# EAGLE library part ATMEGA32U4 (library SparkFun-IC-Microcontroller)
Atmel MCU, 32KByte Atmel 44-pin 8-bit Microcontroller with 32KBytes of ISP Flash and USB Controller Datasheet SparkFun Products LilyPad Arduino USB - ATmega32U4 Board (DEV-12049) Pro Micro - 5V/16MHz (DEV-12640) Pro Micro - 3.3V/8MHz (DEV-12587) Fio v3 - ATmega32U4 (DEV-11520) Qduino Mini (DEV-13614) Makey Makey - Standard Kit (WIG-11511) Makey Makey Deluxe Kit (WIG-11519)
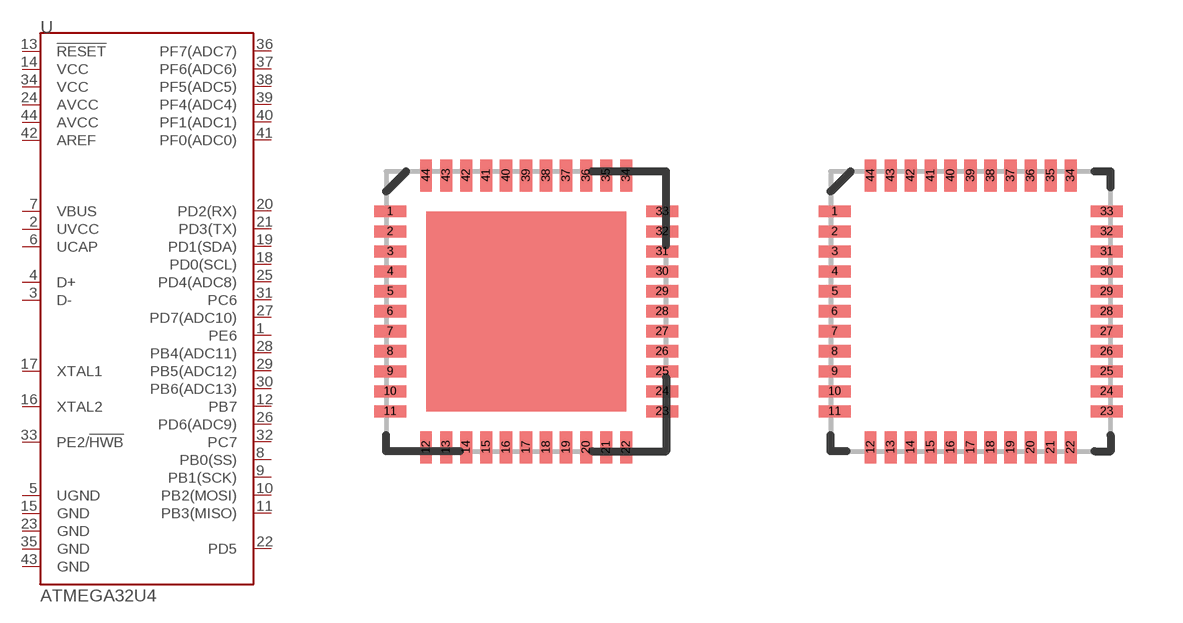
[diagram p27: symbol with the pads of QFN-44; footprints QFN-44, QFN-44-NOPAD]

Designator prefix U

## ATMEGA32U4QFN (PROD_ID: IC-10828; VALUE: 32U4)  [QFN-44]
1  PE6
2  UVCC
3  D-
4  D+
5  UGND
6  UCAP
7  VBUS
8  PB0(SS)
9  PB1(SCK)
10  PB2(MOSI)
11  PB3(MISO)
12  PB7
13  !RESET
14  VCC
15  GND
16  XTAL2
17  XTAL1
18  PD0(SCL)
19  PD1(SDA)
20  PD2(RX)
21  PD3(TX)
22  PD5
23  GND
24  AVCC
25  PD4(ADC8)
26  PD6(ADC9)
27  PD7(ADC10)
28  PB4(ADC11)
29  PB5(ADC12)
30  PB6(ADC13)
31  PC6
32  PC7
33  PE2/!HWB
34  VCC
35  GND
36  PF7(ADC7)
37  PF6(ADC6)
38  PF5(ADC5)
39  PF4(ADC4)
40  PF1(ADC1)
41  PF0(ADC0)
42  AREF
43  GND
44  AVCC

## ATMEGA32U4QFN2 (PROD_ID: IC-10828; VALUE: 32U4)  [QFN-44-NOPAD]
Pads as for QFN-44

## ATMEGA32U41:1 (PROD_ID: IC-10828; VALUE: 32U4)  [QFN-44-NOPAD_1:1]
Pads as for QFN-44

## ATMEGA32U41:1-LESS_PASTE (PROD_ID: IC-10828; VALUE: 32U4)  [QFN-44-NOPAD_1:1-LESS_PASTE]
Pads as for QFN-44

## ATMEGA32U4TQFP-44 (PROD_ID: IC-11161; VALUE: 32U4)  [TQFP44]
Pads as for QFN-44

## ATMEGA32U4QFN3 (PROD_ID: IC-10828; VALUE: 32U4)  [QFN-44-PAD_1:1-LESS_PASTE]
Pads as for QFN-44

## Footprint QFN-44 (pad centres in mm)
smd 0.8 x 0.3: 1 -3.4,2.5; 2 -3.4,2; 3 -3.4,1.5; 4 -3.4,1; 5 -3.4,0.5; 6 -3.4,0; 7 -3.4,-0.5; 8 -3.4,-1; 9 -3.4,-1.5; 10 -3.4,-2; 11 -3.4,-2.5; 23 3.4,-2.5; 24 3.4,-2; 25 3.4,-1.5; 26 3.4,-1; 27 3.4,-0.5; 28 3.4,0; 29 3.4,0.5; 30 3.4,1; 31 3.4,1.5; 32 3.4,2; 33 3.4,2.5
smd 0.3 x 0.8: 12 -2.5,-3.4; 13 -2,-3.4; 14 -1.5,-3.4; 15 -1,-3.4; 16 -0.5,-3.4; 17 0,-3.4; 18 0.5,-3.4; 19 1,-3.4; 20 1.5,-3.4; 21 2,-3.4; 22 2.5,-3.4; 34 2.5,3.4; 35 2,3.4; 36 1.5,3.4; 37 1,3.4; 38 0.5,3.4; 39 0,3.4; 40 -0.5,3.4; 41 -1,3.4; 42 -1.5,3.4; 43 -2,3.4; 44 -2.5,3.4

## Footprint QFN-44-NOPAD (pad centres in mm)
smd 0.8 x 0.3: 1 -3.4,2.5; 2 -3.4,2; 3 -3.4,1.5; 4 -3.4,1; 5 -3.4,0.5; 6 -3.4,0; 7 -3.4,-0.5; 8 -3.4,-1; 9 -3.4,-1.5; 10 -3.4,-2; 11 -3.4,-2.5; 23 3.4,-2.5; 24 3.4,-2; 25 3.4,-1.5; 26 3.4,-1; 27 3.4,-0.5; 28 3.4,0; 29 3.4,0.5; 30 3.4,1; 31 3.4,1.5; 32 3.4,2; 33 3.4,2.5
smd 0.3 x 0.8: 12 -2.5,-3.4; 13 -2,-3.4; 14 -1.5,-3.4; 15 -1,-3.4; 16 -0.5,-3.4; 17 0,-3.4; 18 0.5,-3.4; 19 1,-3.4; 20 1.5,-3.4; 21 2,-3.4; 22 2.5,-3.4; 34 2.5,3.4; 35 2,3.4; 36 1.5,3.4; 37 1,3.4; 38 0.5,3.4; 39 0,3.4; 40 -0.5,3.4; 41 -1,3.4; 42 -1.5,3.4; 43 -2,3.4; 44 -2.5,3.4

## Footprint QFN-44-NOPAD_1:1 (pad centres in mm)
smd 0.8 x 0.3: 1 -3.337,2.458; 2 -3.337,1.958; 3 -3.337,1.479; 4 -3.337,0.979; 5 -3.337,0.5; 6 -3.337,0; 7 -3.337,-0.5; 8 -3.337,-0.979; 9 -3.337,-1.479; 10 -3.337,-1.958; 11 -3.337,-2.458; 23 3.337,-2.458; 24 3.337,-1.958; 25 3.337,-1.479; 26 3.337,-0.979; 27 3.337,-0.5; 28 3.337,0; 29 3.337,0.5; 30 3.337,0.979; 31 3.337,1.479; 32 3.337,1.958; 33 3.337,2.458
smd 0.3 x 0.8: 12 -2.458,-3.337; 13 -1.958,-3.337; 14 -1.479,-3.337; 15 -0.979,-3.337; 16 -0.5,-3.337; 17 0,-3.337; 18 0.5,-3.337; 19 0.979,-3.337; 20 1.479,-3.337; 21 1.958,-3.337; 22 2.458,-3.337; 34 2.458,3.337; 35 1.958,3.337; 36 1.479,3.337; 37 0.979,3.337; 38 0.5,3.337; 39 0,3.337; 40 -0.5,3.337; 41 -0.979,3.337; 42 -1.479,3.337; 43 -1.958,3.337; 44 -2.458,3.337

## Footprint QFN-44-NOPAD_1:1-LESS_PASTE (pad centres in mm)
smd 0.8 x 0.3: 1 -3.337,2.458; 2 -3.337,1.958; 3 -3.337,1.479; 4 -3.337,0.979; 5 -3.337,0.5; 6 -3.337,0; 7 -3.337,-0.5; 8 -3.337,-0.979; 9 -3.337,-1.479; 10 -3.337,-1.958; 11 -3.337,-2.458; 23 3.337,-2.458; 24 3.337,-1.958; 25 3.337,-1.479; 26 3.337,-0.979; 27 3.337,-0.5; 28 3.337,0; 29 3.337,0.5; 30 3.337,0.979; 31 3.337,1.479; 32 3.337,1.958; 33 3.337,2.458
smd 0.3 x 0.8: 12 -2.458,-3.337; 13 -1.958,-3.337; 14 -1.479,-3.337; 15 -0.979,-3.337; 16 -0.5,-3.337; 17 0,-3.337; 18 0.5,-3.337; 19 0.979,-3.337; 20 1.479,-3.337; 21 1.958,-3.337; 22 2.458,-3.337; 34 2.458,3.337; 35 1.958,3.337; 36 1.479,3.337; 37 0.979,3.337; 38 0.5,3.337; 39 0,3.337; 40 -0.5,3.337; 41 -0.979,3.337; 42 -1.479,3.337; 43 -1.958,3.337; 44 -2.458,3.337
